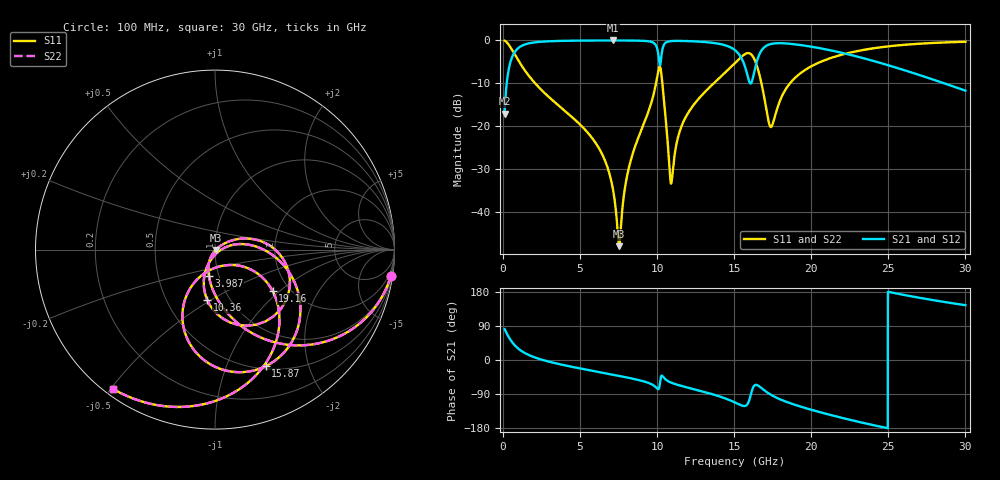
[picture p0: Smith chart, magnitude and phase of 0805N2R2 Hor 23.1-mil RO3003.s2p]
# GHz S MA R 50
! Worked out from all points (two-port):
!   3201 points, 100 MHz to 30 GHz, reference 50 ohm
!   highest |S21| = -0.03 dB at 7.127 GHz (marker M1); lowest = -17.1 dB at 100 MHz (marker M2)
!   |S21| within 3 dB of the highest: 706.9 MHz to 10.06 GHz (9.357 GHz wide, 174 % of centre); 16.66 GHz to 22.12 GHz (5.458 GHz wide, 28.1 % of centre)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
!   lowest |S11| = -48.1 dB at 7.528 GHz (marker M3), VSWR 1.01, Z = 50.3 - j0.278 ohm
!   |S11| at or under -10 dB: 2.071 GHz to 9.925 GHz (7.854 GHz wide, 131 % of centre); 10.33 GHz to 13.68 GHz (3.348 GHz wide, 27.9 % of centre); 16.76 GHz to 18.63 GHz (1.864 GHz wide, 10.5 % of centre)
!   |S22| runs from -48.1 to -0.1 dB; largest |S21 - S12| = 0
!   S11 on the Smith chart (normalised r, x): 100 MHz: 1, -13; 3.987 GHz: 0.90, -0.27; 10.36 GHz: 0.79, -0.48; 15.87 GHz: 0.53, -1.39; 19.16 GHz: 1.64, -0.89; 30 GHz: 0.02, -0.51
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0.1  0.9903 -8.6  0.139 81.4  0.139 81.4  0.9903 -8.6
0.5485  0.7916 -40.8  0.6105 49.2  0.6105 49.2  0.7916 -40.8
1.408125  0.4464 -71.4  0.8937 18.5  0.8937 18.5  0.4464 -71.4
3.987  0.1512 -103.1  0.9862 -13.9  0.9862 -13.9  0.1512 -103.1
5.089563  0.09997 -111.5  0.9922 -23.0  0.9922 -23.0  0.09997 -111.5
6.416375  0.04726 -119.4  0.9955 -33.3  0.9955 -33.3  0.04726 -119.4
7.1265  0.0184 -117.5  0.996 -38.8  0.996 -38.8  0.0184 -117.5
7.528281  0.003945 -44.4  0.9958 -41.9  0.9958 -41.9  0.003945 -44.4
8.182344  0.03354 34.4  0.9943 -47.3  0.9943 -47.3  0.03354 34.4
9.733406  0.221 15.3  0.9425 -66.1  0.9425 -66.1  0.221 15.3
10.06978  0.4389 -19.2  0.6943 -77.0  0.6943 -77.0  0.4389 -19.2
10.35944  0.2846 -98.6  0.8106 -43.1  0.8106 -43.1  0.2846 -98.6
10.92941  0.02189 -35.5  0.9797 -60.1  0.9797 -60.1  0.02189 -35.5
11.92919  0.1343 13.2  0.9799 -72.3  0.9799 -72.3  0.1343 13.2
15.05  0.5437 -30.0  0.7671 -112.1  0.7671 -112.1  0.5437 -30.0
15.87225  0.7082 -66.5  0.3808 -115.8  0.3808 -115.8  0.7082 -66.5
16.52631  0.4668 -112.1  0.6137 -67.0  0.6137 -67.0  0.4668 -112.1
17.36725  0.09717 -77.2  0.905 -91.4  0.905 -91.4  0.09717 -77.2
19.16125  0.3947 -35.7  0.8875 -121.1  0.8875 -121.1  0.3947 -35.7
20.03956  0.5014 -44.6  0.8402 -131.8  0.8402 -131.8  0.5014 -44.6
25.01978  0.8506 -91.4  0.5096 179.6  0.5096 179.6  0.8506 -91.4
30  0.9617 -126.1  0.2585 144.6  0.2585 144.6  0.9617 -126.1
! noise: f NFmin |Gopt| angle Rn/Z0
0.1  0.0009625  0.9384  1.445  0.003485
3.417  0.00629  0.7036  20.08  0.004039
6.743  0.01131  0.685  37.89  0.006255
10.06  0.127  0.953  55.14  0.4777
13.39  0.03356  0.7906  71.18  0.02201
16.7  0.1637  0.9437  87.12  0.3418
20.03  0.05349  0.8131  100.9  0.02458
23.35  0.05489  0.7974  113.5  0.01734
26.67  0.06685  0.8168  125.8  0.01645
30  0.088  0.85  138  0.01679
